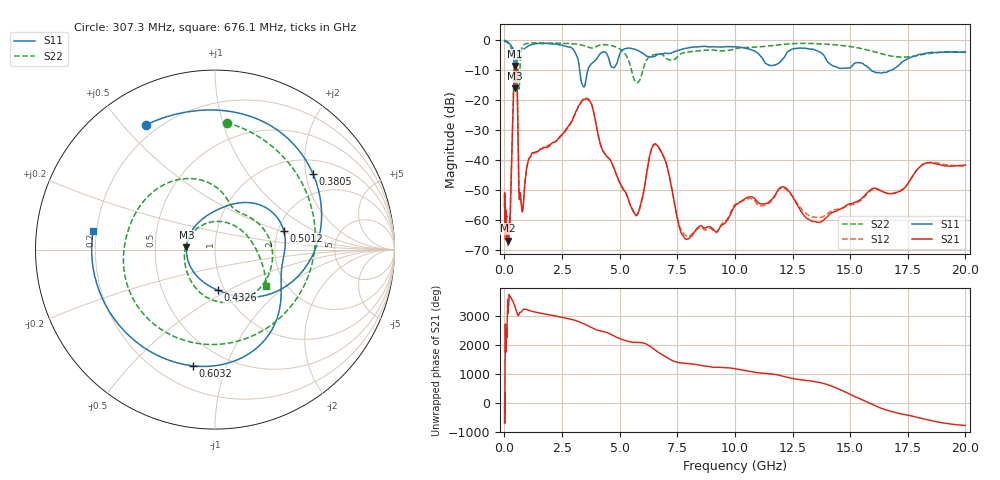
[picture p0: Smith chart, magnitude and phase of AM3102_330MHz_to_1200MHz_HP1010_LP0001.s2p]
! Date/Time: Tue, Sep 11, 2018 5:18 PM
! Network Analyzer: Agilent Technologies E8362B Rev: A.07.50.63
! Sweep from 0.010 to 20.000 GHz, 1601 Points, Sweep Type: LOG
! Power Supply: 4.949 V, 0.001 A
# Hz S DB R 50
!freq MagS11 AngS11 MagS21 AngS21 MagS12 AngS12 MagS22 AngS22
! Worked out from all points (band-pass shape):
!   1601 points, 10 MHz to 20 GHz, reference 50 ohm
!   highest |S21| = -8.55 dB at 473.4 MHz (marker M1); lowest = -66.9 dB at 167.3 MHz (marker M2)
!   |S21| within 3 dB of the highest: 424 MHz to 538.4 MHz (114.4 MHz wide, 23.8 % of centre)
!   lowest |S11| = -16.0 dB at 449.3 MHz (marker M3), VSWR 1.38, Z = 36.3 + j0.955 ohm
!   |S11| at or under -10 dB: 425.5 MHz to 476.6 MHz (51.08 MHz wide, 11.3 % of centre); 3.266 GHz to 3.619 GHz (353.1 MHz wide, 10.3 % of centre); 15.91 GHz to 16.76 GHz (846.3 MHz wide, 5.18 % of centre)
!   |S22| runs from -16.2 to -0.2 dB; largest |S21 - S12| = 0.0054
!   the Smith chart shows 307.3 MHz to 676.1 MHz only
!   S11 on the Smith chart (normalised r, x): 307.3 MHz: 0.15, +0.58; 380.5 MHz: 1.37, +2.20; 432.6 MHz: 0.93, -0.44; 501.2 MHz: 2.15, +0.54; 603.2 MHz: 0.34, -0.77; 676.1 MHz: 0.19, +0.07
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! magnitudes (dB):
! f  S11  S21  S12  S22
! 10 MHz  0.0  -54.3  -52.1  -0.2
! 35.55 MHz  0.0  -63.9  -64.2  -0.3
! 126.4 MHz  -0.4  -64.0  -66.4  -0.7
! 167.3 MHz  -0.6  -66.9  -68.4  -0.9
! 307.3 MHz  -2.0  -43.0  -43.1  -3.0
! 380.5 MHz  -3.2  -21.0  -21.0  -5.6
! 432.6 MHz  -12.9  -10.4  -10.5  -5.7
! 447.2 MHz  -15.9  -9.2  -9.2  -6.1
! 449.3 MHz  -16.0  -9.1  -9.1  -6.1
! 473.4 MHz  -10.7  -8.5  -8.6  -6.5
! 501.2 MHz  -8.0  -8.8  -8.8  -8.3
! 551.2 MHz  -6.8  -14.4  -14.4  -11.6
! 603.2 MHz  -3.6  -36.9  -37.1  -10.9
! 676.1 MHz  -3.3  -51.4  -51.5  -9.1
! 1.59 GHz  -1.0  -36.3  -36.3  -0.8
! 3.617 GHz  -10.1  -19.7  -19.5  -2.2
! 5.652 GHz  -2.9  -57.9  -58.2  -13.5
! 6.549 GHz  -5.2  -34.6  -34.8  -4.7
! 7.92 GHz  -2.5  -66.5  -65.4  -3.9
! 12.03 GHz  -6.6  -49.0  -49.3  -1.4
! 13.68 GHz  -3.9  -60.9  -59.2  -1.1
! 20 GHz  -3.9  -41.6  -42.1  -3.8
